TYPE ST_Parameter_HomeParaCoE :
STRUCT
	HomeMethod			: SINT;	(* 回零方法 *)
    Acceleration		: LREAL;(* 回零中加速度 *)
    VelocityForSwitch	: LREAL;(* 回零一段速度 *)
    VelocityForIndex	: LREAL;(* 回零二段速度 *)
    HomeOffset			: LREAL;(* 回零偏置 *)
END_STRUCT
END_TYPE
